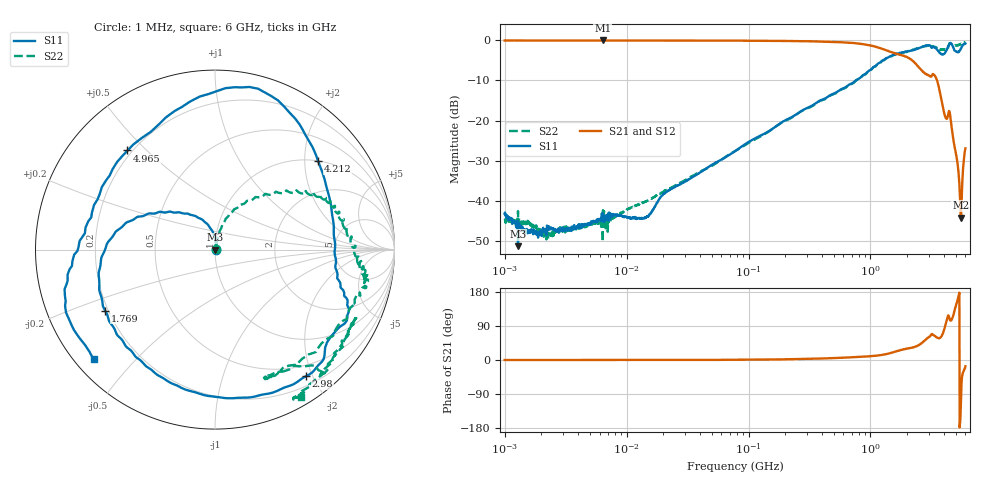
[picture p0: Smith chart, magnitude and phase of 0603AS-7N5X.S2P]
!s-Parameter Generated by FASTRON Sdn. Bhd.
!FASTRON P/N : 0603AS-7N5X
!Keysight Technologies: E5071C_MY46733604_B.14.02
!Date: Thu Nov 30 10:38:47 2023
!Version  :Rev01  Thu Nov 30 10:38:47 2023
!Data & Calibration Information:
!Freq  S11:SOLT2(ON)  S21:SOLT2(ON)  S12:SOLT2(ON)  S22:SOLT2(ON)
!PortZ  Port1:50+j0  Port2:50+j0
!When reading reference impedance value at option line is always used.
! Remarks : This data is being provided solely for informational purposes.
# Hz S dB R 50
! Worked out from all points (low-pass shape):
!   1601 points, 1 MHz to 6 GHz, reference 50 ohm
!   highest |S21| = -0.03 dB at 6.378 MHz (marker M1); lowest = -44.2 dB at 5.496 GHz (marker M2)
!   |S21| within 3 dB of the highest: start of sweep to 1.513 GHz
!   lowest |S11| = -51.3 dB at 1.288 MHz (marker M3), VSWR 1.01, Z = 50.3 - j0.0935 ohm
!   |S11| at or under -10 dB: start of sweep to 757.2 MHz
!   |S22| runs from -50.2 to -0.5 dB; largest |S21 - S12| = 0.0053
!   S11 on the Smith chart (normalised r, x): 1 MHz: 1.01, +0.00; 1.769 GHz: 0.19, -0.25; 2.98 GHz: 0.33, -1.91; 4.212 GHz: 1.01, +2.33; 4.965 GHz: 0.18, +0.44; 6 GHz: 0.05, -0.38
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1000000  -43.25 4.5  -0.04 0.0  -0.05 0.0  -44.45 7.3
1287650  -51.29 -20.0  -0.06 0.0  -0.02 0.1  -42.56 -2.2
2190642  -47.19 20.3  -0.04 0.0  -0.04 0.0  -48.34 29.3
4277066  -46.71 33.0  -0.05 -0.0  -0.05 0.0  -46.68 33.4
6378092  -45.10 51.5  -0.03 -0.1  -0.05 -0.1  -50.24 36.8
1.391995e7  -44.22 64.4  -0.04 0.0  -0.06 0.0  -40.37 48.4
1.823719e7  -39.93 66.4  -0.05 0.0  -0.06 0.1  -38.34 59.8
7.757876e7  -27.62 85.2  -0.08 0.5  -0.09 0.5  -27.59 75.0
3.307917e8  -16.28 107.8  -0.24 3.2  -0.25 3.2  -16.44 72.8
9.600186e8  -7.68 150.8  -1.18 9.5  -1.18 9.4  -7.71 48.1
1.414819e9  -4.15 -178.4  -2.71 17.1  -2.72 17.0  -4.21 29.5
1.769228e9  -3.10 -151.0  -3.61 26.4  -3.62 26.2  -3.21 22.4
2.365139e9  -2.18 -109.9  -5.88 35.7  -5.90 35.7  -2.21 -1.1
2.687444e9  -1.57 -82.0  -7.82 46.8  -7.84 46.9  -1.52 -9.6
2.98045e9  -1.22 -54.3  -8.73 59.4  -8.73 59.5  -1.26 -12.5
3.401721e9  -1.89 -23.1  -9.01 62.7  -9.00 62.6  -1.75 -28.8
3.867453e9  -3.53 -1.1  -15.77 65.9  -15.77 65.8  -2.20 -66.3
4.211689e9  -2.42 40.6  -19.55 104.5  -19.54 104.3  -2.31 -62.2
4.573027e9  -0.76 80.6  -20.30 104.0  -20.31 103.8  -0.91 -45.7
4.964745e9  -2.66 131.4  -27.42 138.6  -27.43 138.5  -1.25 -28.3
5.496363e9  -2.10 -177.9  -44.16 -126.2  -44.14 -126.5  -0.89 -43.7
6e9  -0.80 -137.9  -26.91 -16.6  -26.89 -16.8  -0.45 -59.6
